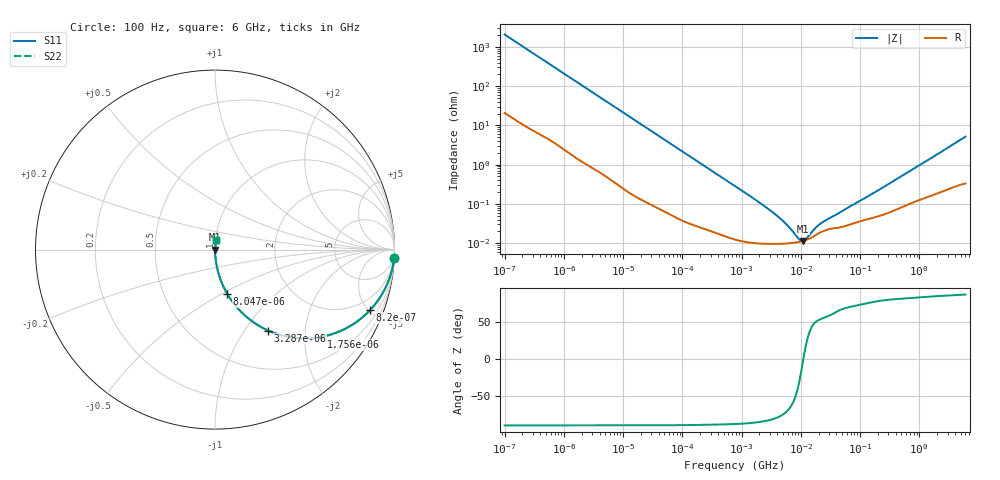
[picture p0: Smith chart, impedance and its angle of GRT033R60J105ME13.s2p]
!Murata Part Number: GRT033R60J105ME13
!These Parameters are Measured in Series Mode Connection
!Data Generated on Jun 19, 2026
!  o--ll--o
!Port1  Port2
!  o------o
!Operation Temp=25[degC], DC Bias Voltage=0[V]
!Freq. Start=100[Hz] Stop=6[GHz] 401[Steps]
# Hz S RI R 50
!Freq.(Hz) S11(Real) S11(Imag) S21(Real) S21(Imag) S12(Real) S12(Imag) S22(Real) S22(Imag)
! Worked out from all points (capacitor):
!   401 points, 100 Hz to 6 GHz, reference 50 ohm
!   read as one part in series: C = 766 nF near 109 Hz
!   lowest |Z| = 11.4 mohm at 10.87 MHz (marker M1)
!   series resonance near 11.04 MHz, so ESL is about 270 pH
!   S11 on the Smith chart (normalised r, x): 100 Hz: 1, -41; 820 Hz: 1.06, -5.13; 1.756 kHz: 1.03, -2.41; 3.287 kHz: 1.02, -1.29; 8.047 kHz: 1.01, -0.53; 6 GHz: 1.01, +0.10
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100  0.9972 -0.0481  0.0028 0.0481  0.0028 0.0481  0.9972 -0.0481
293  0.9793 -0.1373  0.0207 0.1373  0.0207 0.1373  0.9793 -0.1373
524  0.9387 -0.2341  0.0613 0.2341  0.0613 0.2341  0.9387 -0.2341
820  0.8651 -0.3358  0.1349 0.3358  0.1349 0.3358  0.8651 -0.3358
1174  0.7611 -0.4207  0.2389 0.4207  0.2389 0.4207  0.7611 -0.4207
1756  0.5909 -0.4861  0.4091 0.4861  0.4091 0.4861  0.5909 -0.4861
2008  0.526 -0.4937  0.474 0.4937  0.474 0.4937  0.526 -0.4937
3287  0.2968 -0.451  0.7032 0.451  0.7032 0.451  0.2968 -0.451
5143  0.1496 -0.3508  0.8504 0.3508  0.8504 0.3508  0.1496 -0.3508
8047  0.0685 -0.2469  0.9315 0.2469  0.9315 0.2469  0.0685 -0.2469
17227  0.0167 -0.1225  0.9833 0.1225  0.9833 0.1225  0.0167 -0.1225
40335  0.00361 -0.0534  0.9964 0.0534  0.9964 0.0534  0.00361 -0.0534
774597  0.000132 -0.00286  0.9999 0.00286  0.9999 0.00286  0.000132 -0.00286
3712478  9.61e-05 -0.000534  0.9999 0.000534  0.9999 0.000534  9.61e-05 -0.000534
5809218  9.84e-05 -0.000278  0.9999 0.000278  0.9999 0.000278  9.84e-05 -0.000278
9090158  0.000107 -7.89e-05  0.9999 7.89e-05  0.9999 7.89e-05  0.000107 -7.89e-05
1.087309e7  0.000114 -6.2e-06  0.9999 6.2e-06  0.9999 6.2e-06  0.000114 -6.2e-06
1.243624e7  0.000122 4.76e-05  0.9999 -4.76e-05  0.9999 -4.76e-05  0.000122 4.76e-05
1.555665e7  0.000142 0.000137  0.9999 -0.000137  0.9999 -0.000137  0.000142 0.000137
2.434276e7  0.000205 0.000292  0.9998 -0.000292  0.9998 -0.000292  0.000205 0.000292
3.124326e8  0.000615 0.00325  0.9994 -0.00325  0.9994 -0.00325  0.000615 0.00325
6e9  0.00593 0.0511  0.9941 -0.0511  0.9941 -0.0511  0.00593 0.0511
